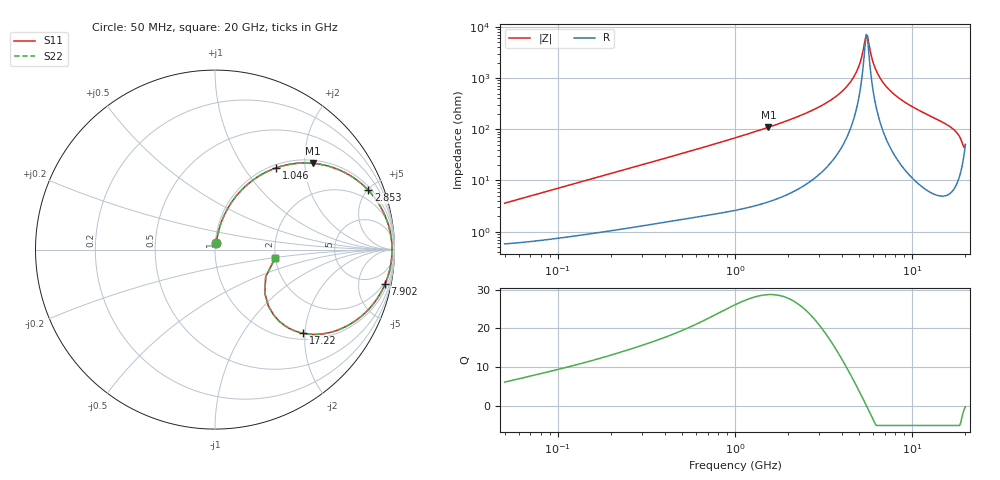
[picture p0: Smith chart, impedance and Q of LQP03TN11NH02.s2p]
!Murata Part Number: LQP03TN11NH02
!These Parameters are Measured in Series Mode Connection
!  o--[Z]--o
!Port1  Port2
!  o-------o
!Freq. Start=50[MHz] Stop=20[GHz], 401[Steps]
# Hz S RI R 50
!Freq.(Hz) S11(Real) S11(Imag) S21(Real) S21(Imag) S12(Real) S12(Imag) S22(Real) S22(Imag)
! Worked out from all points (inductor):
!   401 points, 50 MHz to 20 GHz, reference 50 ohm
!   read as one part in series: L = 11.2 nH near 51.52 MHz
!   highest Q = 28.7 at 1.544 GHz (marker M1), where L = 11.3 nH
!   self-resonance near 5.516 GHz
!   S11 on the Smith chart (normalised r, x): 50 MHz: 1.01, +0.07; 1.046 GHz: 1.05, +1.42; 2.853 GHz: 1.23, +5.05; 7.902 GHz: 1.65, -9.70; 17.22 GHz: 1.13, -1.96; 20 GHz: 1.99, -0.21
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5e7  0.00696 0.0351  0.993 -0.0351  0.993 -0.0351  0.00696 0.0351
1.364002e8  0.0171 0.092  0.9829 -0.092  0.9829 -0.092  0.0171 0.092
3.721004e8  0.0711 0.2294  0.9289 -0.2294  0.9289 -0.2294  0.0711 0.2294
6.285508e8  0.1622 0.3461  0.8378 -0.3461  0.8378 -0.3461  0.1622 0.3461
1e9  0.3217 0.4483  0.6783 -0.4483  0.6783 -0.4483  0.3217 0.4483
1.045961e9  0.3418 0.4558  0.6582 -0.4558  0.6582 -0.4558  0.3418 0.4558
1.544007e9  0.5432 0.481  0.4568 -0.481  0.4568 -0.481  0.5432 0.481
2.728004e9  0.8354 0.3497  0.1646 -0.3497  0.1646 -0.3497  0.8354 0.3497
2.853386e9  0.8535 0.3316  0.1465 -0.3316  0.1465 -0.3316  0.8535 0.3316
3.736399e9  0.9388 0.2075  0.0612 -0.2075  0.0612 -0.2075  0.9388 0.2075
4.472136e9  0.9721 0.1149  0.0279 -0.1149  0.0279 -0.1149  0.9721 0.1149
4.966507e9  0.9825 0.0589  0.0175 -0.0589  0.0175 -0.0589  0.9825 0.0589
5.515528e9  0.9863 0.00212  0.0137 -0.00212  0.0137 -0.00212  0.9863 0.00212
5.683258e9  0.9862 -0.0142  0.0138 0.0142  0.0138 0.0142  0.9862 -0.0142
6.034176e9  0.9843 -0.0468  0.0157 0.0468  0.0157 0.0468  0.9843 -0.0468
6.311513e9  0.9814 -0.0713  0.0186 0.0713  0.0186 0.0713  0.9814 -0.0713
7.442007e9  0.9598 -0.1602  0.0402 0.1602  0.0402 0.1602  0.9598 -0.1602
7.901521e9  0.9476 -0.192  0.0524 0.192  0.0524 0.192  0.9476 -0.192
1.257102e10  0.7645 -0.4084  0.2355 0.4084  0.2355 0.4084  0.7645 -0.4084
1.721783e10  0.4925 -0.4668  0.5075 0.4668  0.5075 0.4668  0.4925 -0.4668
1.855685e10  0.36 -0.4009  0.64 0.4009  0.64 0.4009  0.36 -0.4009
2e10  0.3352 -0.047  0.6648 0.047  0.6648 0.047  0.3352 -0.047
